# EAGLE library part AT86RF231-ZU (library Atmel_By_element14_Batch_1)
Low Power 2.4 GHz Transceiver for ZigBee
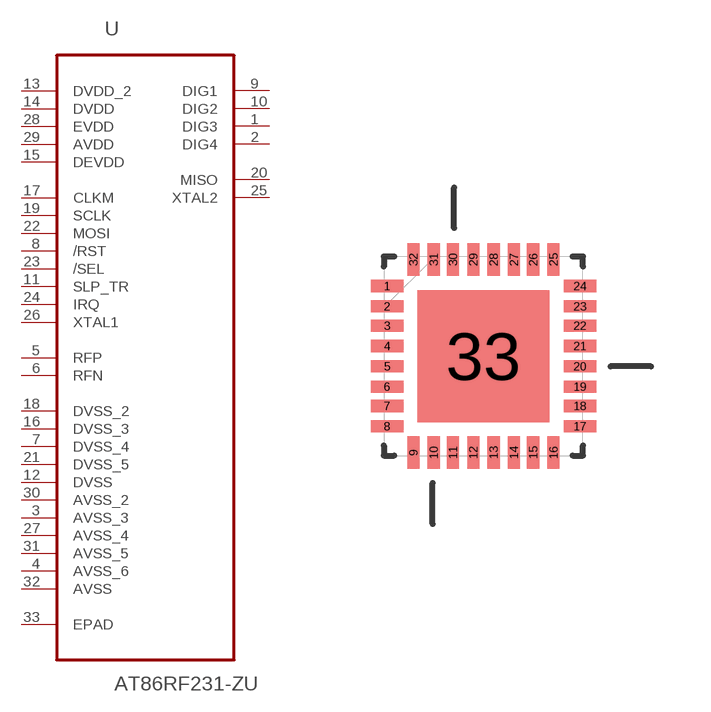
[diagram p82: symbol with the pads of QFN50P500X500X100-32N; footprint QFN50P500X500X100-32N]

Designator prefix U

## AT86RF231-ZU (DESCRIPTION: Low Power 2.4 GHz Transceiver for ZigBee; MPN: AT86RF231-ZU; OC_FARNELL: 1748493; OC_NEWARK: -; PACKAGE: QFN-32; SUPPLIER: ATMEL)  [QFN50P500X500X100-32N]
1  DIG3  out
2  DIG4  out
3  AVSS_3  pwr
4  AVSS_6  pwr
5  RFP  in
6  RFN  in
7  DVSS_4  pwr
8  /RST  in
9  DIG1  out
10  DIG2  out
11  SLP_TR  in
12  DVSS  pwr
13  DVDD_2  pwr
14  DVDD  pwr
15  DEVDD  pwr
16  DVSS_3  pwr
17  CLKM  in
18  DVSS_2  pwr
19  SCLK  in
20  MISO  out
21  DVSS_5  pwr
22  MOSI  in
23  /SEL  in
24  IRQ  in
25  XTAL2  out
26  XTAL1  in
27  AVSS_4  pwr
28  EVDD  pwr
29  AVDD  pwr
30  AVSS_2  pwr
31  AVSS_5  pwr
32  AVSS  pwr
33  EPAD  pas

## Footprint QFN50P500X500X100-32N (pad centres in mm)
smd 0.813 x 0.305: 1 -2.413,1.753; 2 -2.413,1.245; 3 -2.413,0.762; 4 -2.413,0.254; 5 -2.413,-0.254; 6 -2.413,-0.762; 7 -2.413,-1.245; 8 -2.413,-1.753; 17 2.413,-1.753; 18 2.413,-1.245; 19 2.413,-0.762; 20 2.413,-0.254; 21 2.413,0.254; 22 2.413,0.762; 23 2.413,1.245; 24 2.413,1.753
smd 0.305 x 0.813: 9 -1.753,-2.413; 10 -1.245,-2.413; 11 -0.762,-2.413; 12 -0.254,-2.413; 13 0.254,-2.413; 14 0.762,-2.413; 15 1.245,-2.413; 16 1.753,-2.413; 25 1.753,2.413; 26 1.245,2.413; 27 0.762,2.413; 28 0.254,2.413; 29 -0.254,2.413; 30 -0.762,2.413; 31 -1.245,2.413; 32 -1.753,2.413
smd 3.302 x 3.302: 33 0,0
